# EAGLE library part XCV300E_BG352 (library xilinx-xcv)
xcv300e_bg352 edit this description Auto generated by make-symbol-device-package-bsdl.ulp Rev. 26 Source: xcv300e_bg352.bsd
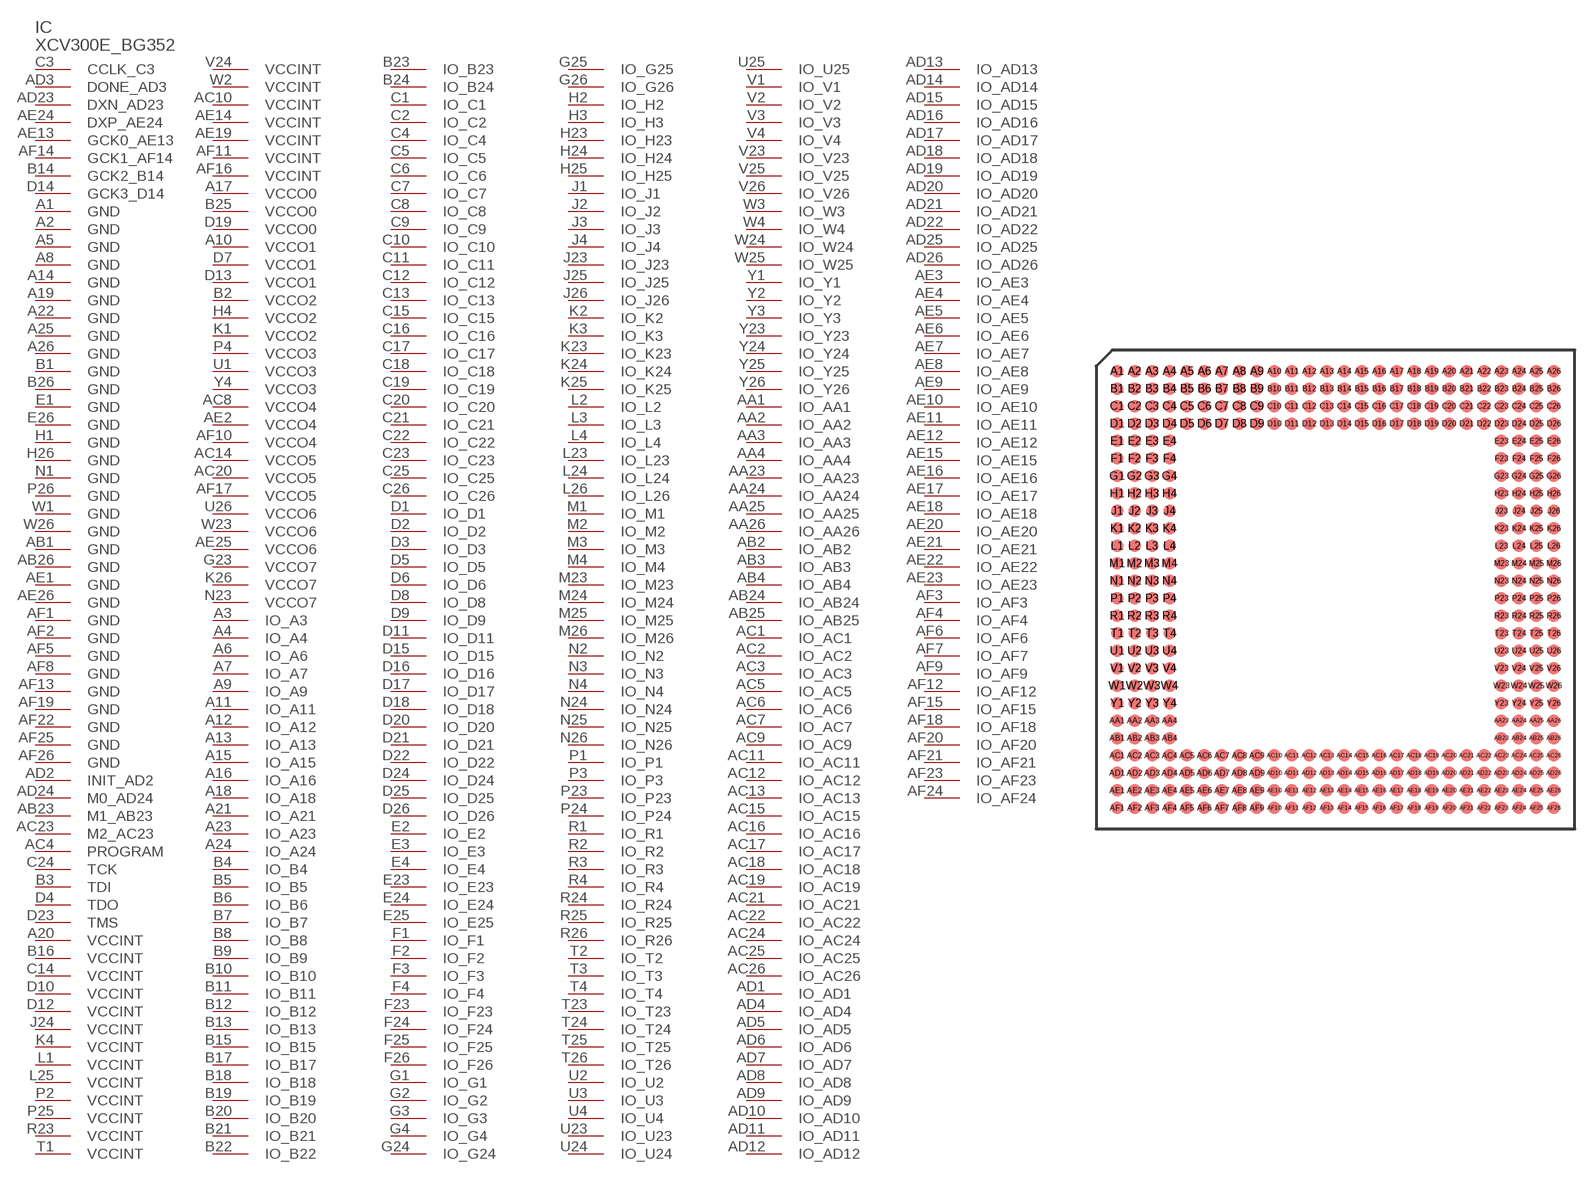
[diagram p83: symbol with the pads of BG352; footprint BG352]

Designator prefix IC

## XCV300E_BG352 (OC_FARNELL: unknown; OC_NEWARK: unknown)  [BG352]
A1  GND  pwr
A2  GND  pwr
A3  IO_A3
A4  IO_A4
A5  GND  pwr
A6  IO_A6
A7  IO_A7
A8  GND  pwr
A9  IO_A9
A10  VCCO1  pwr
A11  IO_A11
A12  IO_A12
A13  IO_A13
A14  GND  pwr
A15  IO_A15
A16  IO_A16
A17  VCCO0  pwr
A18  IO_A18
A19  GND  pwr
A20  VCCINT  pwr
A21  IO_A21
A22  GND  pwr
A23  IO_A23
A24  IO_A24
A25  GND  pwr
A26  GND  pwr
AA1  IO_AA1
AA2  IO_AA2
AA3  IO_AA3
AA4  IO_AA4
AA23  IO_AA23
AA24  IO_AA24
AA25  IO_AA25
AA26  IO_AA26
AB1  GND  pwr
AB2  IO_AB2
AB3  IO_AB3
AB4  IO_AB4
AB23  M1_AB23  in
AB24  IO_AB24
AB25  IO_AB25
AB26  GND  pwr
AC1  IO_AC1
AC2  IO_AC2
AC3  IO_AC3
AC4  PROGRAM  in
AC5  IO_AC5
AC6  IO_AC6
AC7  IO_AC7
AC8  VCCO4  pwr
AC9  IO_AC9
AC10  VCCINT  pwr
AC11  IO_AC11
AC12  IO_AC12
AC13  IO_AC13
AC14  VCCO5  pwr
AC15  IO_AC15
AC16  IO_AC16
AC17  IO_AC17
AC18  IO_AC18
AC19  IO_AC19
AC20  VCCO5  pwr
AC21  IO_AC21
AC22  IO_AC22
AC23  M2_AC23  in
AC24  IO_AC24
AC25  IO_AC25
AC26  IO_AC26
AD1  IO_AD1
AD2  INIT_AD2
AD3  DONE_AD3
AD4  IO_AD4
AD5  IO_AD5
AD6  IO_AD6
AD7  IO_AD7
AD8  IO_AD8
AD9  IO_AD9
AD10  IO_AD10
AD11  IO_AD11
AD12  IO_AD12
AD13  IO_AD13
AD14  IO_AD14
AD15  IO_AD15
AD16  IO_AD16
AD17  IO_AD17
AD18  IO_AD18
AD19  IO_AD19
AD20  IO_AD20
AD21  IO_AD21
AD22  IO_AD22
AD23  DXN_AD23  pas
AD24  M0_AD24  in
AD25  IO_AD25
AD26  IO_AD26
AE1  GND  pwr
AE2  VCCO4  pwr
AE3  IO_AE3
AE4  IO_AE4
AE5  IO_AE5
AE6  IO_AE6
AE7  IO_AE7
AE8  IO_AE8
AE9  IO_AE9
AE10  IO_AE10
AE11  IO_AE11
AE12  IO_AE12
AE13  GCK0_AE13  in
AE14  VCCINT  pwr
AE15  IO_AE15
AE16  IO_AE16
AE17  IO_AE17
AE18  IO_AE18
AE19  VCCINT  pwr
AE20  IO_AE20
AE21  IO_AE21
AE22  IO_AE22
AE23  IO_AE23
AE24  DXP_AE24  pas
AE25  VCCO6  pwr
AE26  GND  pwr
AF1  GND  pwr
AF2  GND  pwr
AF3  IO_AF3
AF4  IO_AF4
AF5  GND  pwr
AF6  IO_AF6
AF7  IO_AF7
AF8  GND  pwr
AF9  IO_AF9
AF10  VCCO4  pwr
AF11  VCCINT  pwr
AF12  IO_AF12
AF13  GND  pwr
AF14  GCK1_AF14  in
AF15  IO_AF15
AF16  VCCINT  pwr
AF17  VCCO5  pwr
AF18  IO_AF18
AF19  GND  pwr
AF20  IO_AF20
AF21  IO_AF21
AF22  GND  pwr
AF23  IO_AF23
AF24  IO_AF24
AF25  GND  pwr
AF26  GND  pwr
B1  GND  pwr
B2  VCCO2  pwr
B3  TDI  in
B4  IO_B4
B5  IO_B5
B6  IO_B6
B7  IO_B7
B8  IO_B8
B9  IO_B9
B10  IO_B10
B11  IO_B11
B12  IO_B12
B13  IO_B13
B14  GCK2_B14  in
B15  IO_B15
B16  VCCINT  pwr
B17  IO_B17
B18  IO_B18
B19  IO_B19
B20  IO_B20
B21  IO_B21
B22  IO_B22
B23  IO_B23
B24  IO_B24
B25  VCCO0  pwr
B26  GND  pwr
C1  IO_C1
C2  IO_C2
C3  CCLK_C3
C4  IO_C4
C5  IO_C5
C6  IO_C6
C7  IO_C7
C8  IO_C8
C9  IO_C9
C10  IO_C10
C11  IO_C11
C12  IO_C12
C13  IO_C13
C14  VCCINT  pwr
C15  IO_C15
C16  IO_C16
C17  IO_C17
C18  IO_C18
C19  IO_C19
C20  IO_C20
C21  IO_C21
C22  IO_C22
C23  IO_C23
C24  TCK  in
C25  IO_C25
C26  IO_C26
D1  IO_D1
D2  IO_D2
D3  IO_D3
D4  TDO  out
D5  IO_D5
D6  IO_D6
D7  VCCO1  pwr
D8  IO_D8
D9  IO_D9
D10  VCCINT  pwr
D11  IO_D11
D12  VCCINT  pwr
D13  VCCO1  pwr
D14  GCK3_D14  in
D15  IO_D15
D16  IO_D16
D17  IO_D17
D18  IO_D18
D19  VCCO0  pwr
D20  IO_D20
D21  IO_D21
D22  IO_D22
D23  TMS  in
D24  IO_D24
D25  IO_D25
D26  IO_D26
E1  GND  pwr
E2  IO_E2
E3  IO_E3
E4  IO_E4
E23  IO_E23
E24  IO_E24
E25  IO_E25
E26  GND  pwr
F1  IO_F1
F2  IO_F2
F3  IO_F3
F4  IO_F4
F23  IO_F23
F24  IO_F24
F25  IO_F25
F26  IO_F26
G1  IO_G1
G2  IO_G2
G3  IO_G3
G4  IO_G4
G23  VCCO7  pwr
G24  IO_G24
G25  IO_G25
G26  IO_G26
H1  GND  pwr
H2  IO_H2
H3  IO_H3
H4  VCCO2  pwr
H23  IO_H23
H24  IO_H24
H25  IO_H25
H26  GND  pwr
J1  IO_J1
J2  IO_J2
J3  IO_J3
J4  IO_J4
J23  IO_J23
J24  VCCINT  pwr
J25  IO_J25
J26  IO_J26
K1  VCCO2  pwr
K2  IO_K2
K3  IO_K3
K4  VCCINT  pwr
K23  IO_K23
K24  IO_K24
K25  IO_K25
K26  VCCO7  pwr
L1  VCCINT  pwr
L2  IO_L2
L3  IO_L3
L4  IO_L4
L23  IO_L23
L24  IO_L24
L25  VCCINT  pwr
L26  IO_L26
M1  IO_M1
M2  IO_M2
M3  IO_M3
M4  IO_M4
M23  IO_M23
M24  IO_M24
M25  IO_M25
M26  IO_M26
N1  GND  pwr
N2  IO_N2
N3  IO_N3
N4  IO_N4
N23  VCCO7  pwr
N24  IO_N24
N25  IO_N25
N26  IO_N26
P1  IO_P1
P2  VCCINT  pwr
P3  IO_P3
P4  VCCO3  pwr
P23  IO_P23
P24  IO_P24
P25  VCCINT  pwr
P26  GND  pwr
R1  IO_R1
R2  IO_R2
R3  IO_R3
R4  IO_R4
R23  VCCINT  pwr
R24  IO_R24
R25  IO_R25
R26  IO_R26
T1  VCCINT  pwr
T2  IO_T2
T3  IO_T3
T4  IO_T4
T23  IO_T23
T24  IO_T24
T25  IO_T25
T26  IO_T26
U1  VCCO3  pwr
U2  IO_U2
U3  IO_U3
U4  IO_U4
U23  IO_U23
U24  IO_U24
U25  IO_U25
U26  VCCO6  pwr
V1  IO_V1
V2  IO_V2
V3  IO_V3
V4  IO_V4
V23  IO_V23
V24  VCCINT  pwr
V25  IO_V25
V26  IO_V26
W1  GND  pwr
W2  VCCINT  pwr
W3  IO_W3
W4  IO_W4
W23  VCCO6  pwr
W24  IO_W24
W25  IO_W25
W26  GND  pwr
Y1  IO_Y1
Y2  IO_Y2
Y3  IO_Y3
Y4  VCCO3  pwr
Y23  IO_Y23
Y24  IO_Y24
Y25  IO_Y25
Y26  IO_Y26

## Footprint BG352 (pad centres in mm)
xcv100e_bg352 edit this description Auto generated by make-symbol-device-package-bsdl.ulp Rev. 26 Source: xcv100e_bg352.bsd
smd 0.9 x 0.9: A1 -15.875,15.875; A2 -14.605,15.875; A3 -13.335,15.875; A4 -12.065,15.875; A5 -10.795,15.875; A6 -9.525,15.875; A7 -8.255,15.875; A8 -6.985,15.875; A9 -5.715,15.875; A10 -4.445,15.875; A11 -3.175,15.875; A12 -1.905,15.875; A13 -0.635,15.875; A14 0.635,15.875; A15 1.905,15.875; A16 3.175,15.875; A17 4.445,15.875; A18 5.715,15.875; A19 6.985,15.875; A20 8.255,15.875; A21 9.525,15.875; A22 10.795,15.875; A23 12.065,15.875; A24 13.335,15.875; A25 14.605,15.875; A26 15.875,15.875; AA1 -15.875,-9.525; AA2 -14.605,-9.525; AA3 -13.335,-9.525; AA4 -12.065,-9.525; AA23 12.065,-9.525; AA24 13.335,-9.525; AA25 14.605,-9.525; AA26 15.875,-9.525; AB1 -15.875,-10.795; AB2 -14.605,-10.795; AB3 -13.335,-10.795; AB4 -12.065,-10.795; AB23 12.065,-10.795; AB24 13.335,-10.795; AB25 14.605,-10.795; AB26 15.875,-10.795; AC1 -15.875,-12.065; AC2 -14.605,-12.065; AC3 -13.335,-12.065; AC4 -12.065,-12.065; AC5 -10.795,-12.065; AC6 -9.525,-12.065; AC7 -8.255,-12.065; AC8 -6.985,-12.065; AC9 -5.715,-12.065; AC10 -4.445,-12.065; AC11 -3.175,-12.065; AC12 -1.905,-12.065; AC13 -0.635,-12.065; AC14 0.635,-12.065; AC15 1.905,-12.065; AC16 3.175,-12.065; AC17 4.445,-12.065; AC18 5.715,-12.065; AC19 6.985,-12.065; AC20 8.255,-12.065; AC21 9.525,-12.065; AC22 10.795,-12.065; AC23 12.065,-12.065; AC24 13.335,-12.065; AC25 14.605,-12.065; AC26 15.875,-12.065; AD1 -15.875,-13.335; AD2 -14.605,-13.335; AD3 -13.335,-13.335; AD4 -12.065,-13.335; AD5 -10.795,-13.335; AD6 -9.525,-13.335; AD7 -8.255,-13.335; AD8 -6.985,-13.335; AD9 -5.715,-13.335; AD10 -4.445,-13.335; AD11 -3.175,-13.335; AD12 -1.905,-13.335; AD13 -0.635,-13.335; AD14 0.635,-13.335; AD15 1.905,-13.335; AD16 3.175,-13.335; AD17 4.445,-13.335; AD18 5.715,-13.335; AD19 6.985,-13.335; AD20 8.255,-13.335; AD21 9.525,-13.335; AD22 10.795,-13.335; AD23 12.065,-13.335; AD24 13.335,-13.335; AD25 14.605,-13.335; AD26 15.875,-13.335; AE1 -15.875,-14.605; AE2 -14.605,-14.605; AE3 -13.335,-14.605; AE4 -12.065,-14.605; AE5 -10.795,-14.605; AE6 -9.525,-14.605; AE7 -8.255,-14.605; AE8 -6.985,-14.605; AE9 -5.715,-14.605; AE10 -4.445,-14.605; AE11 -3.175,-14.605; AE12 -1.905,-14.605; AE13 -0.635,-14.605; AE14 0.635,-14.605; AE15 1.905,-14.605; AE16 3.175,-14.605; AE17 4.445,-14.605; AE18 5.715,-14.605; AE19 6.985,-14.605; AE20 8.255,-14.605; AE21 9.525,-14.605; AE22 10.795,-14.605; AE23 12.065,-14.605; AE24 13.335,-14.605; AE25 14.605,-14.605; AE26 15.875,-14.605; AF1 -15.875,-15.875; AF2 -14.605,-15.875; AF3 -13.335,-15.875; AF4 -12.065,-15.875; AF5 -10.795,-15.875; AF6 -9.525,-15.875; AF7 -8.255,-15.875; AF8 -6.985,-15.875; AF9 -5.715,-15.875; AF10 -4.445,-15.875; AF11 -3.175,-15.875; AF12 -1.905,-15.875; AF13 -0.635,-15.875; AF14 0.635,-15.875; AF15 1.905,-15.875; AF16 3.175,-15.875; AF17 4.445,-15.875; AF18 5.715,-15.875; AF19 6.985,-15.875; AF20 8.255,-15.875; AF21 9.525,-15.875; AF22 10.795,-15.875; AF23 12.065,-15.875; AF24 13.335,-15.875; AF25 14.605,-15.875; AF26 15.875,-15.875; B1 -15.875,14.605; B2 -14.605,14.605; B3 -13.335,14.605; B4 -12.065,14.605; B5 -10.795,14.605; B6 -9.525,14.605; B7 -8.255,14.605; B8 -6.985,14.605; B9 -5.715,14.605; B10 -4.445,14.605; B11 -3.175,14.605; B12 -1.905,14.605; B13 -0.635,14.605; B14 0.635,14.605; B15 1.905,14.605; B16 3.175,14.605; B17 4.445,14.605; B18 5.715,14.605; B19 6.985,14.605; B20 8.255,14.605; B21 9.525,14.605; B22 10.795,14.605; B23 12.065,14.605; B24 13.335,14.605; B25 14.605,14.605; B26 15.875,14.605; C1 -15.875,13.335; C2 -14.605,13.335; C3 -13.335,13.335; C4 -12.065,13.335; C5 -10.795,13.335; C6 -9.525,13.335; C7 -8.255,13.335; C8 -6.985,13.335; C9 -5.715,13.335; C10 -4.445,13.335; C11 -3.175,13.335; C12 -1.905,13.335; C13 -0.635,13.335; C14 0.635,13.335; C15 1.905,13.335; C16 3.175,13.335; C17 4.445,13.335; C18 5.715,13.335; C19 6.985,13.335; C20 8.255,13.335; C21 9.525,13.335; C22 10.795,13.335; C23 12.065,13.335; C24 13.335,13.335; C25 14.605,13.335; C26 15.875,13.335; D1 -15.875,12.065; D2 -14.605,12.065; D3 -13.335,12.065; D4 -12.065,12.065; D5 -10.795,12.065; D6 -9.525,12.065; D7 -8.255,12.065; D8 -6.985,12.065; D9 -5.715,12.065; D10 -4.445,12.065; D11 -3.175,12.065; D12 -1.905,12.065; D13 -0.635,12.065; D14 0.635,12.065; D15 1.905,12.065; D16 3.175,12.065; D17 4.445,12.065; D18 5.715,12.065; D19 6.985,12.065; D20 8.255,12.065; D21 9.525,12.065; D22 10.795,12.065; D23 12.065,12.065; D24 13.335,12.065; D25 14.605,12.065; D26 15.875,12.065; E1 -15.875,10.795; E2 -14.605,10.795; E3 -13.335,10.795; E4 -12.065,10.795; E23 12.065,10.795; E24 13.335,10.795; E25 14.605,10.795; E26 15.875,10.795; F1 -15.875,9.525; F2 -14.605,9.525; F3 -13.335,9.525; F4 -12.065,9.525; F23 12.065,9.525; F24 13.335,9.525; F25 14.605,9.525; F26 15.875,9.525; G1 -15.875,8.255; G2 -14.605,8.255; G3 -13.335,8.255; G4 -12.065,8.255; G23 12.065,8.255; G24 13.335,8.255; G25 14.605,8.255; G26 15.875,8.255; H1 -15.875,6.985; H2 -14.605,6.985; H3 -13.335,6.985; H4 -12.065,6.985; H23 12.065,6.985; H24 13.335,6.985; H25 14.605,6.985; H26 15.875,6.985; J1 -15.875,5.715; J2 -14.605,5.715; J3 -13.335,5.715; J4 -12.065,5.715; J23 12.065,5.715; J24 13.335,5.715; J25 14.605,5.715; J26 15.875,5.715; K1 -15.875,4.445; K2 -14.605,4.445; K3 -13.335,4.445; K4 -12.065,4.445; K23 12.065,4.445; K24 13.335,4.445; K25 14.605,4.445; K26 15.875,4.445; L1 -15.875,3.175; L2 -14.605,3.175; L3 -13.335,3.175; L4 -12.065,3.175; L23 12.065,3.175; L24 13.335,3.175; L25 14.605,3.175; L26 15.875,3.175; M1 -15.875,1.905; M2 -14.605,1.905; M3 -13.335,1.905; M4 -12.065,1.905; M23 12.065,1.905; M24 13.335,1.905; M25 14.605,1.905; M26 15.875,1.905; N1 -15.875,0.635; N2 -14.605,0.635; N3 -13.335,0.635; N4 -12.065,0.635; N23 12.065,0.635; N24 13.335,0.635; N25 14.605,0.635; N26 15.875,0.635; P1 -15.875,-0.635; P2 -14.605,-0.635; P3 -13.335,-0.635; P4 -12.065,-0.635; P23 12.065,-0.635; P24 13.335,-0.635; P25 14.605,-0.635; P26 15.875,-0.635; R1 -15.875,-1.905; R2 -14.605,-1.905; R3 -13.335,-1.905; R4 -12.065,-1.905; R23 12.065,-1.905; R24 13.335,-1.905; R25 14.605,-1.905; R26 15.875,-1.905; T1 -15.875,-3.175; T2 -14.605,-3.175; T3 -13.335,-3.175; T4 -12.065,-3.175; T23 12.065,-3.175; T24 13.335,-3.175; T25 14.605,-3.175; T26 15.875,-3.175; U1 -15.875,-4.445; U2 -14.605,-4.445; U3 -13.335,-4.445; U4 -12.065,-4.445; U23 12.065,-4.445; U24 13.335,-4.445; U25 14.605,-4.445; U26 15.875,-4.445; V1 -15.875,-5.715; V2 -14.605,-5.715; V3 -13.335,-5.715; V4 -12.065,-5.715; V23 12.065,-5.715; V24 13.335,-5.715; V25 14.605,-5.715; V26 15.875,-5.715; W1 -15.875,-6.985; W2 -14.605,-6.985; W3 -13.335,-6.985; W4 -12.065,-6.985; W23 12.065,-6.985; W24 13.335,-6.985; W25 14.605,-6.985; W26 15.875,-6.985; Y1 -15.875,-8.255; Y2 -14.605,-8.255; Y3 -13.335,-8.255; Y4 -12.065,-8.255; Y23 12.065,-8.255; Y24 13.335,-8.255; Y25 14.605,-8.255; Y26 15.875,-8.255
